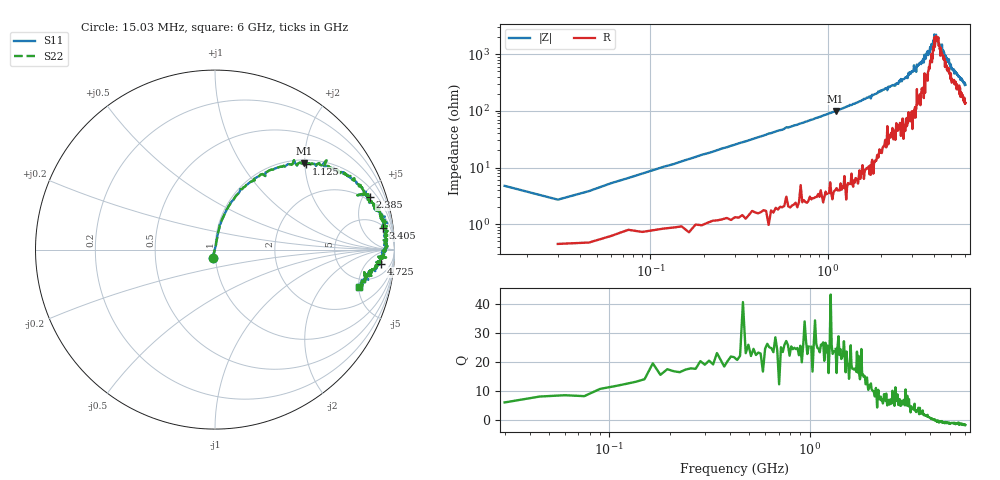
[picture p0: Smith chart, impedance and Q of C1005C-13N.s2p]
!	Network	Analyzer	HP8753E.07.74:	Oct	30	2002	Serial	No.	JP38451487
!	Hewlett-Packard
!	7	Sep	2009	8:44:59
!	Frequency	S11	S21	S12	S22
#	HZ	S	RI	R	50
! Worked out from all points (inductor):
!   400 points, 15.03 MHz to 6 GHz, reference 50 ohm
!   read as one part in series: L = 13.8 nH near 45.03 MHz
!   highest Q = 26.1 at 1.11 GHz (marker M1), where L = 14.2 nH
!   self-resonance near 4.164 GHz
!   S11 on the Smith chart (normalised r, x): 15.03 MHz: 0.97, -0.09; 1.125 GHz: 1.09, +2.02; 2.385 GHz: 1.65, +5.60; 3.405 GHz: 6, +13; 4.725 GHz: 11, -13; 6 GHz: 3.75, -5.04
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1.502992e7  -0.0133 -0.0467  1.01 0.0467  1.01 0.0467  -0.0133 -0.0467
3.002985e7  0.00536 0.0265  0.995 -0.0265  0.995 -0.0265  0.00536 0.0265
1.200294e8  0.0185 0.101  0.981 -0.101  0.981 -0.101  0.0185 0.101
3.150284e8  0.0767 0.243  0.923 -0.243  0.923 -0.243  0.0767 0.243
1.020025e9  0.449 0.478  0.551 -0.478  0.551 -0.478  0.449 0.478
1.110024e9  0.496 0.48  0.504 -0.48  0.504 -0.48  0.496 0.48
1.125024e9  0.506 0.479  0.494 -0.479  0.494 -0.479  0.506 0.479
2.01002e9  0.812 0.349  0.188 -0.349  0.188 -0.349  0.812 0.349
2.385018e9  0.862 0.292  0.138 -0.292  0.138 -0.292  0.862 0.292
3.015015e9  0.946 0.184  0.0544 -0.184  0.0544 -0.184  0.946 0.184
3.405013e9  0.937 0.119  0.0634 -0.119  0.0634 -0.119  0.937 0.119
3.855011e9  0.955 0.0452  0.045 -0.0452  0.045 -0.0452  0.955 0.0452
3.91501e9  0.94 0.0531  0.0596 -0.0531  0.0596 -0.0531  0.94 0.0531
4.00501e9  0.961 0.0192  0.0388 -0.0192  0.0388 -0.0192  0.961 0.0192
4.03501e9  0.942 0.0258  0.058 -0.0258  0.058 -0.0258  0.942 0.0258
4.09501e9  0.959 0.0139  0.0412 -0.0139  0.0412 -0.0139  0.959 0.0139
4.335008e9  0.934 -0.045  0.0657 0.045  0.0657 0.045  0.934 -0.045
4.425008e9  0.953 -0.0439  0.0472 0.0439  0.0472 0.0439  0.953 -0.0439
4.455008e9  0.922 -0.0354  0.0781 0.0354  0.0781 0.0354  0.922 -0.0354
4.725006e9  0.925 -0.08  0.0753 0.08  0.0753 0.08  0.925 -0.08
5.010005e9  0.887 -0.106  0.113 0.106  0.113 0.106  0.887 -0.106
6e9  0.802 -0.21  0.198 0.21  0.198 0.21  0.802 -0.21
